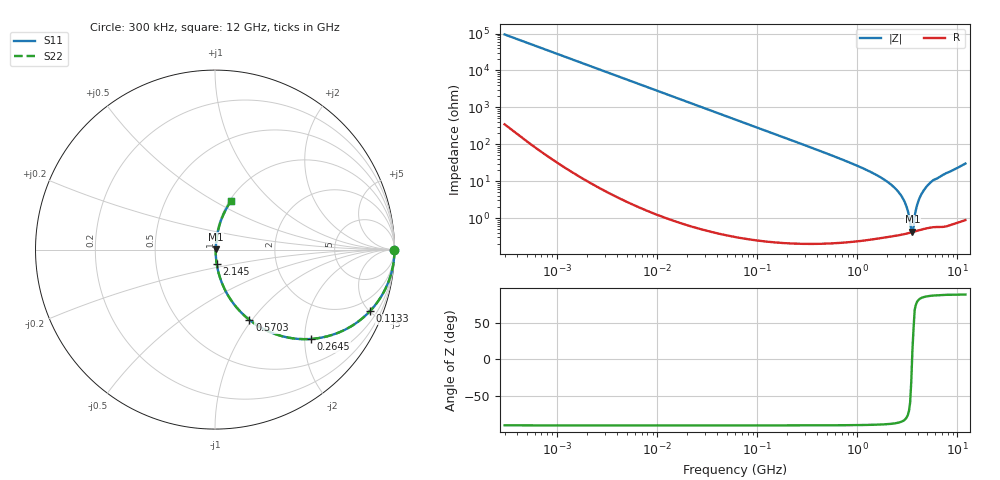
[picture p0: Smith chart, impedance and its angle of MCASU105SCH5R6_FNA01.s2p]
! MCASU105SCH5R6_FNA01  S-PARAMETER MODEL  ( Standard Model )
! Model Generated by TAIYO YUDEN Corporation (http://www.ty-top.com)
! Version 1.0
! TAIYO YUDEN Control No. 230609
! Copyright(c) 2023 TAIYO YUDEN CO.,LTD. All Rights Reserved.
! Product Description (link to TY-COMPAS)
! https://ds.yuden.co.jp/TYCOMPAS/or/detail?pn=MCASU105SCH5R6DFNA01&u=M
! Products Name : Multilayer Ceramic Capacitors
! Characteristics :
!  Capacitance : 5.6 [pF] , Rated Voltage : 50 [V] , TCC : CH / C0H
!  Case Size : 1.0 x 0.5 / 0.039 x 0.02 [mm/inch] , Thickness : 0.5 / 0.02 [mm/inch]
!  (Conditions: Temperature = 25 [degC] , DC Bias Voltage = 0 [V])
! External Node Assignments :
!  1  o---| |---o  2
! GND o---------o GND
! Frequency Range : 0.3MHz  -  12000MHz  [ 401 STEP ]
# MHZ S RI R 50
! Freq[MHz].  S11 Real  S11 Imag  S21 Real  S21 Imag  S12 Real  S12 Imag  S22 Real  S22 Imag
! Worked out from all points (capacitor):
!   401 points, 300 kHz to 12 GHz, reference 50 ohm
!   read as one part in series: C = 5.6 pF near 316.3 kHz
!   lowest |Z| = 424 mohm at 3.548 GHz (marker M1)
!   series resonance near 3.523 GHz, so ESL is about 360 pH
!   S11 on the Smith chart (normalised r, x): 300 kHz: open; 113.3 MHz: 1.00, -5.01; 264.5 MHz: 1.00, -2.14; 570.3 MHz: 1.00, -0.97; 2.145 GHz: 1.01, -0.17; 12 GHz: 1.02, +0.60
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0.3  1 -0.00106  4.98e-06 0.00106  4.98e-06 0.00106  1 -0.00106
1.769972  1 -0.00623  4.35e-05 0.00623  4.35e-05 0.00623  1 -0.00623
10.44266  0.9986 -0.0367  0.00136 0.0367  0.00136 0.0367  0.9986 -0.0367
60  0.9572 -0.2021  0.0428 0.2021  0.0428 0.2021  0.9572 -0.2021
113.3117  0.8624 -0.344  0.1376 0.344  0.1376 0.344  0.8624 -0.344
264.5085  0.533 -0.498  0.467 0.498  0.467 0.498  0.533 -0.498
353.9943  0.3873 -0.4859  0.6127 0.4859  0.6127 0.4859  0.3873 -0.4859
570.2811  0.1916 -0.3914  0.8084 0.3914  0.8084 0.3914  0.1916 -0.3914
1229.528  0.0417 -0.1938  0.9583 0.1938  0.9583 0.1938  0.0417 -0.1938
2088.533  0.0107 -0.0866  0.9893 0.0866  0.9893 0.0866  0.0107 -0.0866
2144.601  0.0099 -0.0819  0.9901 0.0819  0.9901 0.0819  0.0099 -0.0819
2514.07  0.00634 -0.0544  0.9937 0.0544  0.9937 0.0544  0.00634 -0.0544
2870.14  0.00466 -0.0324  0.9953 0.0324  0.9953 0.0324  0.00466 -0.0324
3107.553  0.00416 -0.0195  0.9958 0.0195  0.9958 0.0195  0.00416 -0.0195
3454.93  0.00406 -0.00242  0.9959 0.00242  0.9959 0.00242  0.00406 -0.00242
3547.679  0.00414 0.000861  0.9959 -0.000861  0.9959 -0.000861  0.00414 0.000861
3642.919  0.00423 0.00381  0.9958 -0.00381  0.9958 -0.00381  0.00423 0.00381
3944.255  0.00495 0.0215  0.9951 -0.0215  0.9951 -0.0215  0.00495 0.0215
4158.869  0.00576 0.033  0.9942 -0.033  0.9942 -0.033  0.00576 0.033
5006.236  0.0109 0.0742  0.9891 -0.0742  0.9891 -0.0742  0.0109 0.0742
5868.704  0.0174 0.1075  0.9826 -0.1075  0.9826 -0.1075  0.0174 0.1075
12000  0.0893 0.271  0.9107 -0.271  0.9107 -0.271  0.0893 0.271
